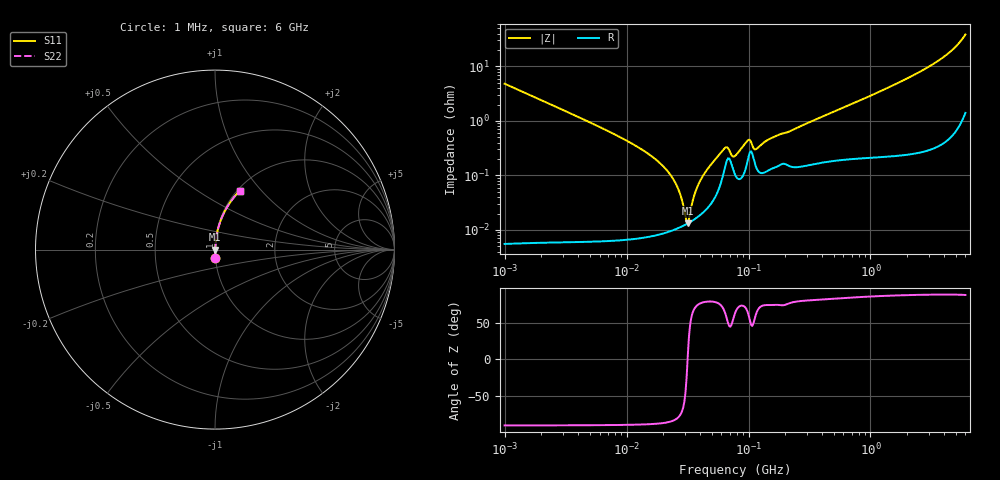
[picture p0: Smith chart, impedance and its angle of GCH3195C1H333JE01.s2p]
!Murata Part Number: GCH3195C1H333JE01
!These Parameters are Measured in Series Mode Connection
!Data Generated on Mar 13, 2026
!  o--ll--o
!Port1  Port2
!  o------o
!Operation Temp=25[degC], DC Bias Voltage=0[V]
!Freq. Start=1000[kHz] Stop=6[GHz] 401[Steps]
# Hz S RI R 50
!Freq.(Hz) S11(Real) S11(Imag) S21(Real) S21(Imag) S12(Real) S12(Imag) S22(Real) S22(Imag)
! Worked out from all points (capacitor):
!   401 points, 1 MHz to 6 GHz, reference 50 ohm
!   read as one part in series: C = 33 nF near 1.044 MHz
!   lowest |Z| = 13.2 mohm at 31.76 MHz (marker M1)
!   series resonance near 31.65 MHz, so ESL is about 770 pH
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1000000  0.00237 -0.0481  0.9976 0.0481  0.9976 0.0481  0.00237 -0.0481
4293785  0.000182 -0.011  0.9998 0.011  0.9998 0.011  0.000182 -0.011
1.093935e7  8.22e-05 -0.00389  0.9999 0.00389  0.9999 0.00389  8.22e-05 -0.00389
1.843659e7  8.49e-05 -0.00174  0.9999 0.00174  0.9999 0.00174  8.49e-05 -0.00174
2.499862e7  0.000103 -0.000739  0.9999 0.000739  0.9999 0.000739  0.000103 -0.000739
2.787038e7  0.000113 -0.000398  0.9999 0.000398  0.9999 0.000398  0.000113 -0.000398
3.040356e7  0.000125 -0.000126  0.9999 0.000126  0.9999 0.000126  0.000125 -0.000126
3.175522e7  0.000132 1.03e-05  0.9999 -1.03e-05  0.9999 -1.03e-05  0.000132 1.03e-05
3.245342e7  0.000135 7.89e-05  0.9999 -7.89e-05  0.9999 -7.89e-05  0.000135 7.89e-05
3.540316e7  0.000153 0.000357  0.9998 -0.000357  0.9998 -0.000357  0.000153 0.000357
3.779011e7  0.000169 0.000571  0.9998 -0.000571  0.9998 -0.000571  0.000169 0.000571
4.697123e7  0.000266 0.00136  0.9997 -0.00136  0.9997 -0.00136  0.000266 0.00136
6.368941e7  0.00133 0.00286  0.9987 -0.00286  0.9987 -0.00286  0.00133 0.00286
6.652088e7  0.00189 0.00269  0.9981 -0.00269  0.9981 -0.00269  0.00189 0.00269
7.745967e7  0.00104 0.00202  0.999 -0.00202  0.999 -0.00202  0.00104 0.00202
9.83954e7  0.00189 0.00394  0.9981 -0.00394  0.9981 -0.00394  0.00189 0.00394
1.170949e8  0.00132 0.00281  0.9987 -0.00281  0.9987 -0.00281  0.00132 0.00281
1.520136e8  0.00132 0.00459  0.9987 -0.00459  0.9987 -0.00459  0.00132 0.00459
3.325952e8  0.00168 0.0098  0.9983 -0.0098  0.9983 -0.0098  0.00168 0.0098
1.428092e9  0.00395 0.0415  0.9961 -0.0415  0.9961 -0.0415  0.00395 0.0415
3.5601e9  0.0186 0.1224  0.9814 -0.1224  0.9814 -0.1224  0.0186 0.1224
6e9  0.1384 0.3276  0.8616 -0.3276  0.8616 -0.3276  0.1384 0.3276
